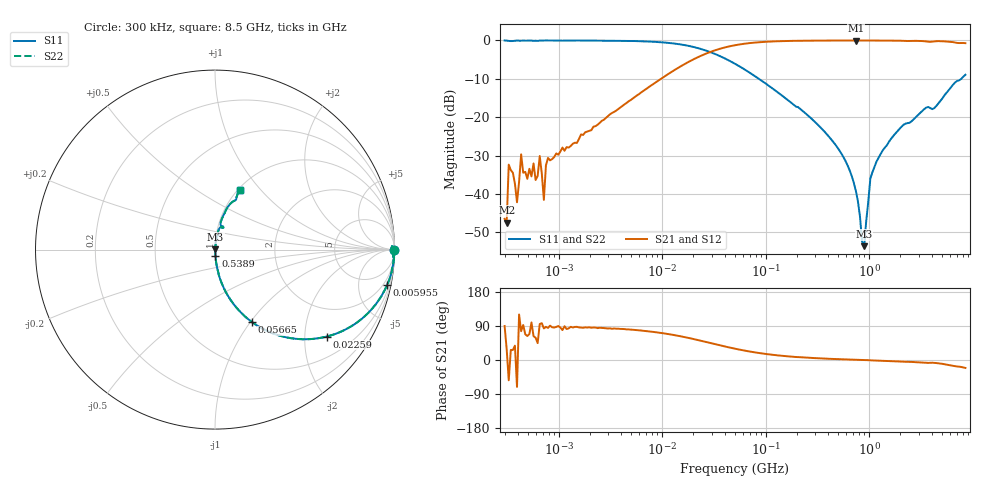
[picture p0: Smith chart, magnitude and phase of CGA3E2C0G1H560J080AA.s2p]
! S-parameter Generated by TDK Corporation
! Copyright(C) 2015 TDK Corporation.
! All Rights Reserved.
! TDK P/N: CGA3E2C0G1H560J080AA (Multilayer Ceramic Chip Capacitors)
! Property: C=56pF
! Size(LxWxT): 1.6x0.8x0.8mm, 0.063x0.031x0.031inches
! Model Type: s2p (Touchstone File Format Version 1.0)
! Frequency: DC=Yes Start=0.3MHz Stop=8500MHz 225points Log-sweep
! Note:
! Model Generated on Jun. 23, 2015
! Hash(MD5):
! Port Assignments:
!  1 ---| |--- 2
! Applicable Conditions:
!  Temperature = 25 degC
!  DC Bias Voltage = 0 V
!  Small Signal Operation
! Terms and conditions regarding TDK Simulation Models
! (1)This simulation model is being provided solely for informational purposes. Please refer to the specifications of the products in terms of detailed characteristics of such products.
! (2)In no event shall TDK Corporation of any of its subsidiaries be liable for any loss or damage arising, directly or indirectly,
!  From any information contained in this simulation model, including, but not limited to loss or damages arising from any inaccuracies, omissions or errors in connection with such information.
! (3)Any and all copyrights on this simulation model are owned by TDK Corporation.
!  Duplication or redistribution of this simulation model without prior written permission from TDK Corporation is prohibited.
! (4)This simulation model is subject to any modification or change without any prior notice.
! (5)Neither TDK Corporation nor any of its subsidiaries shall make any warranty, express or implied,
!  Including but not limited to the correctness, implied warranties of merchantability and fitness for a particular purpose with respect to this simulation models.
! (6)The use of this simulation model shall be deemed to have consented to the terms and conditions hereof.
# MHz S MA R 50
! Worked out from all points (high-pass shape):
!   224 points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, 300 kHz to 8.5 GHz, reference 50 ohm
!   highest |S21| = -0.01 dB at 743.4 MHz (marker M1); lowest = -47.4 dB at 314.1 kHz (marker M2)
!   |S21| within 3 dB of the highest: 29.04 MHz to end of sweep
!   lowest |S11| = -53.6 dB at 893.5 MHz (marker M3), VSWR 1.00, Z = 50.2 + j0.118 ohm
!   |S11| at or under -10 dB: 86.06 MHz to 7.747 GHz (7.661 GHz wide, 196 % of centre)
!   |S22| runs from -53.6 to 0.0 dB; largest |S21 - S12| = 6.5e-13
!   S11 on the Smith chart (normalised r, x): 300 kHz: open; 5.955 MHz: 1.06, -9.80; 22.59 MHz: 1.00, -2.57; 56.65 MHz: 1.00, -1.02; 538.9 MHz: 1.00, -0.07; 8.5 GHz: 1.03, +0.77
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0.3  1 -0.3  0.004754 89.7  0.004754 89.7  1 -0.3
0.3141136  0.9963 -0.1  0.004263 28.7  0.004263 28.7  0.9963 -0.1
0.3288911  0.9858 1.1  0.02419 -53.6  0.02419 -53.6  0.9858 1.1
0.3952884  0.9975 0.4  0.007818 -71.0  0.007818 -71.0  0.9975 0.4
0.4333561  0.9926 -1.8  0.03291 76.0  0.03291 76.0  0.9926 -1.8
0.597865  0.9922 -0.8  0.01525 58.9  0.01525 58.9  0.9922 -0.8
0.6554417  0.9959 -1.8  0.03129 94.9  0.03129 94.9  0.9959 -1.8
0.7185633  0.999 -0.5  0.008393 83.2  0.008393 83.2  0.999 -0.5
0.7877636  0.9977 -1.7  0.02953 84.7  0.02953 84.7  0.9977 -1.7
1.72111  0.9966 -3.4  0.05884 85.0  0.05884 85.0  0.9966 -3.4
5.954923  0.9787 -11.5  0.1997 78.1  0.1997 78.1  0.9787 -11.5
9.430415  0.9508 -18.0  0.3083 71.9  0.3083 71.9  0.9508 -18.0
22.58783  0.7892 -37.9  0.6136 52.1  0.6136 52.1  0.7892 -37.9
51.67171  0.4884 -60.7  0.8719 29.2  0.8719 29.2  0.4884 -60.7
56.64789  0.4544 -62.9  0.8901 27.0  0.8901 27.0  0.4544 -62.9
283.1228  0.09328 -83.8  0.9943 5.4  0.9943 5.4  0.09328 -83.8
538.8791  0.03364 -85.9  0.9981 1.9  0.9981 1.9  0.03364 -85.9
743.4462  0.01096 -81.2  0.9984 0.6  0.9984 0.6  0.01096 -81.2
893.5346  0.002097 34.2  0.9983 -0.1  0.9983 -0.1  0.002097 34.2
1025.67  0.0159 82.1  0.9979 -0.9  0.9979 -0.9  0.0159 82.1
1551.304  0.04789 83.9  0.996 -2.7  0.996 -2.7  0.04789 83.9
8500  0.3574 67.2  0.9222 -20.9  0.9222 -20.9  0.3574 67.2
